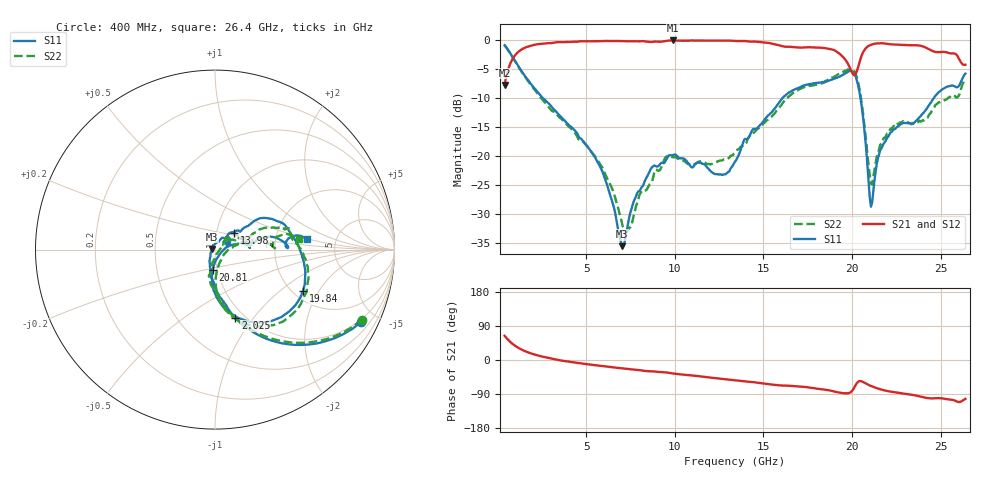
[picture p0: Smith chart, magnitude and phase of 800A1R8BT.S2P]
!  American Technical Ceramics  Date:  12/17/08
!  One Norden Lane
!  Huntington Station,  NY.  11746-2102
!  Tel:  (631) 622-4700  Fax:  (631) 622-4748
!  Part Number  800A1R8BT
!  Description: Broardband capacitor  Mounting Orientation: Vertical
!  Application:
# GHZ S DB R 50
! Freq  |S11|  S11 Ph  |S21|  S21 Ph  |S12|  S12 Ph  |S22|  S22 Ph
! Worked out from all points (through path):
!   401 points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, 400 MHz to 26.4 GHz, reference 50 ohm
!   highest |S21| = 0.00 dB at 9.89 GHz (marker M1); lowest = -7.7 dB at 400 MHz (marker M2)
!   group delay of S21, straight-line fit = 13.7 ps
!   lowest |S11| = -35.5 dB at 7.03 GHz (marker M3), VSWR 1.03, Z = 48.4 + j0.41 ohm
!   |S11| at or under -10 dB: 2.577 GHz to 16.07 GHz (13.49 GHz wide, 145 % of centre); 20.48 GHz to 24.61 GHz (4.128 GHz wide, 18.3 % of centre)
!   |S22| runs from -33.0 to -0.8 dB; largest |S21 - S12| = 0.0096
!   S11 on the Smith chart (normalised r, x): 400 MHz: 0.88, -4.11; 2.025 GHz: 0.91, -0.81; 13.98 GHz: 1.21, +0.23; 19.84 GHz: 2.26, -1.47; 20.81 GHz: 0.95, -0.21; 26.4 GHz: 3.05, +0.49
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0.4  -0.82 -26.2  -7.69 63.8  -7.74 63.9  -0.85 -25.6
1.18  -4.48 -58.1  -1.96 31.9  -2.00 32.0  -4.55 -57.1
2.025  -8.05 -73.5  -0.79 15.3  -0.83 15.4  -8.27 -74.5
4.755  -17.11 -98.3  -0.14 -9.2  -0.17 -9.0  -17.33 -101.1
5.925  -22.69 -114.4  -0.10 -15.9  -0.11 -15.6  -22.04 -101.6
7.03  -35.55 165.3  -0.11 -22.1  -0.11 -21.8  -31.61 -67.8
7.81  -26.98 70.5  -0.14 -26.0  -0.12 -25.7  -28.68 14.5
9.11  -21.64 49.3  -0.23 -31.6  -0.20 -31.2  -22.51 41.2
9.89  -19.81 37.9  0.00 -35.5  -0.01 -35.1  -20.18 39.2
12.555  -23.12 27.6  -0.01 -49.2  -0.01 -49.1  -20.76 38.2
13.4  -20.95 45.4  -0.08 -53.5  -0.06 -53.5  -19.39 31.0
13.985  -16.99 41.3  -0.10 -56.5  -0.07 -56.5  -18.08 27.2
17.755  -7.45 15.2  -1.19 -73.8  -1.15 -73.9  -7.75 16.4
18.99  -6.61 2.0  -1.67 -83.0  -1.63 -83.3  -6.27 -2.1
19.835  -5.33 -25.1  -4.40 -87.1  -4.36 -87.3  -5.02 -28.3
20.355  -7.89 -71.1  -4.53 -57.2  -4.49 -57.5  -7.34 -70.0
20.81  -19.03 -96.7  -1.25 -62.8  -1.21 -63.1  -17.66 -86.5
21.135  -28.08 -16.4  -0.68 -69.7  -0.64 -70.0  -24.94 -25.8
21.525  -19.69 15.1  -0.51 -76.2  -0.47 -76.6  -18.92 10.5
22.11  -16.26 13.2  -0.64 -82.8  -0.61 -83.2  -15.67 14.1
24.255  -11.63 13.9  -1.36 -100.4  -1.33 -100.9  -13.39 14.4
26.4  -5.74 6.5  -4.20 -102.6  -4.18 -103.2  -6.56 7.2
